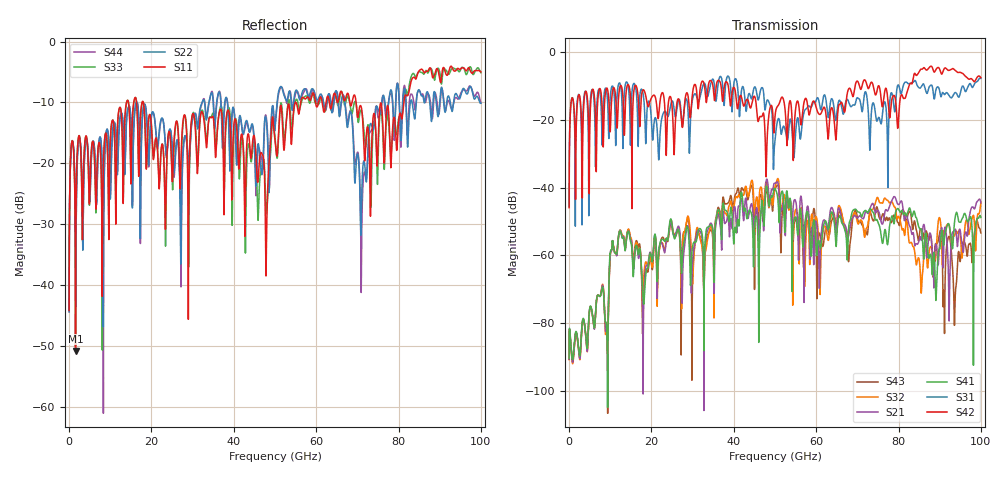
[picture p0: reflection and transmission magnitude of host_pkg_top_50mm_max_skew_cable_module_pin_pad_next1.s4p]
# Hz S RI R 50
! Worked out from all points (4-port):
!   10000 points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, 10 MHz to 100 GHz, reference 50 ohm
!   strongest paths, dB at 10 MHz, 25.01 GHz, 50.01 GHz, 75.01 GHz, 100 GHz:
!     S42: -45.9, -16.0, -18.9, -10.1, -7.5
!     S31: -45.6, -14.3, -26.0, -19.6, -7.7
!     S41: -90.5, -51.2, -40.3, -50.3, -48.8
!     S21: -90.7, -51.8, -38.7, -46.7, -44.5
!     S32: -90.9, -51.7, -39.7, -43.1, -44.3
!     S43: -90.6, -50.9, -40.4, -47.1, -53.4
!   lowest |S11| = -50.8 dB at 1.57 GHz (marker M1), VSWR 1.01, Z = 50.3 - j0.0229 ohm
!   |S11| at or under -10 dB: start of sweep to 13.94 GHz; 18.02 GHz to 54.91 GHz (36.88 GHz wide, 101 % of centre); 69.69 GHz to 81.28 GHz (11.59 GHz wide, 15.3 % of centre)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
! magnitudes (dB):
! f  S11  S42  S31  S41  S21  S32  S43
! 10 MHz  -44.2  -45.9  -45.6  -90.5  -90.7  -90.9  -90.6
! 1.57 GHz  -50.8  -43.5  -32.6  -82.8  -83.3  -83.6  -83.2
! 42.29 GHz  -17.6  -15.6  -10.3  -45.7  -48.9  -42.3  -40.7
! 76.99 GHz  -12.4  -10.7  -16.7  -54.1  -46.5  -43.5  -49.0
! 85.56 GHz  -4.5  -4.9  -10.1  -52.3  -55.6  -70.7  -52.5
! 93.7 GHz  -4.8  -5.3  -11.9  -49.2  -52.4  -53.9  -74.7
! 100 GHz  -5.0  -7.5  -7.7  -48.8  -44.5  -44.3  -53.4
